FUNCTION_BLOCK FileExample03_Trajectory //1x1 1 xbot - DeleteTrajectory, SaveTrajectory, ReadTrajectoryHash. Trajectory file 'TrajectoryDemo.txt' must be on disc in the DemoFilesFolder.  
VAR_INPUT
	Execute : BOOL;
	DemoFilesFolder : STRING(255);	//Folder that contains the GCodeDemo.txt file
END_VAR
VAR_OUTPUT
	Done : BOOL;
END_VAR
VAR_IN_OUT
	PM_Controller : PMControllerType;	// the planar motor controller to use
END_VAR
VAR
	Read_file : ReadFileOnDisk;
	TrajData : ARRAY[0..499999] OF SINT;
	PMC_XYMotion1 : PMC_XYMotion;
	PMC_DeleteTrajectory1 : PMC_DeleteTrajectory;
	PMC_DeactivateXbots1 : PMC_DeactivateXbots;
	PMC_SaveTrajectory1 : PMC_SaveTrajectory;
	PMC_Activatexbots1 : PMC_ActivateXbots;
	PMC_ReadTrajectoryHash1 : PMC_ReadTrajectoryHash;
	xbotID_array12 : ARRAY[0..11] OF USINT;
	trajID_array12 : ARRAY[0..11] OF USINT;
	PMC_ActivateTrajectory1 : PMC_ActivateTrajectory;
END_VAR

//1x1 1 xbot - DeleteTrajectory, SaveTrajectory, ReadTrajectoryHash. Trajectory file 'TrajectoryDemo.txt' must be on disc in the DemoFilesFolder.  

//read trajectory file from disk
Read_file(Execute := Execute,file_path := CONCAT(STR1 := DemoFilesFolder,STR2 := '\TrajectoryDemo.txt'),buffer_size := 500000,data := TrajData);

//delete all trajectories from PMC
PMC_DeleteTrajectory1(Execute := Read_file.Done,TrajID := 0,PM_Controller := PM_Controller);

//deactivate PMC to allow uploading trajectory files
PMC_Deactivatexbots1(Execute := PMC_DeleteTrajectory1.Done,PM_Controller := PM_Controller);

//transfer trajectory file to PMC as trajectory 1
PMC_SaveTrajectory1(Execute := PMC_Deactivatexbots1.Done,TrajID := 1,nBytes := Read_file.file_size,Axises := 63,TimeInterval := 0.010,Bytes := TrajData,PM_Controller := PM_Controller);

//reactivate PMC after uploading the trajectory
PMC_Activatexbots1(Execute := PMC_SaveTrajectory1.Done,PM_Controller := PM_Controller);

//read the MD5 hash of trajectory 1 (should be 0x900D5E503988125A0FB99E7CB3ADFB86)
PMC_ReadTrajectoryHash1(Execute := PMC_Activatexbots1.Done,TrajID := 1,PM_Controller := PM_Controller);

//move xbot to starting position
PMC_XYMotion1(Execute := PMC_ReadTrajectoryHash1.Valid,cmdLB := 0,XbotID := 1,Mode := 0,Type_ := 0,PosX := 0.12,PosY := 0.12,EndVel := 0,MaxVel := 1.0,MaxAcc := 10.0,PM_Controller := PM_Controller);

//xbot 1 runs trajectory 1
xbotID_array12[0] := 1;
trajID_array12[0] := 1;
PMC_ActivateTrajectory1(Execute := PMC_XYMotion1.Done,cmdLB := 0,nXbots := 1,XbotID := xbotID_array12,TrajID := trajID_array12,PM_Controller := PM_Controller);
Done := PMC_ActivateTrajectory1.Done;

END_FUNCTION_BLOCK
